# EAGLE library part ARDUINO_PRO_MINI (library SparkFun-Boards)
SparkFun Pro Mini Pro Mini compatible footprint. Dimensions: 0.7 x 1.3" PCB Thickness: 0.8mm SparkFun Products: 3.3V/8MHz 5V/16MHz
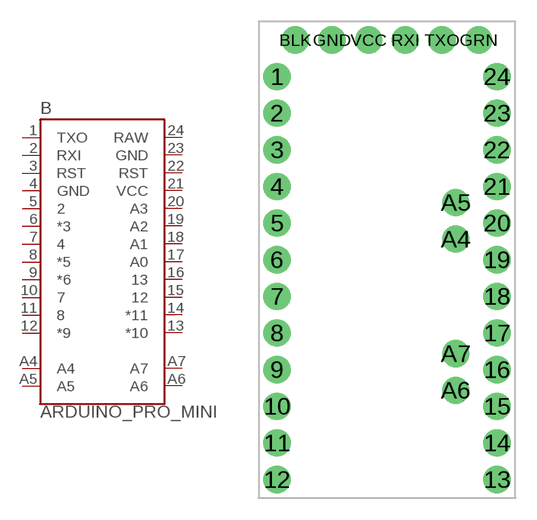
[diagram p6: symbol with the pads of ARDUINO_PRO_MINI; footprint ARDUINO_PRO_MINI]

Designator prefix B

## ARDUINO_PRO_MINI  [ARDUINO_PRO_MINI]
1  TXO
2  RXI
3  RST
4  GND  pwr
5  2
6  *3
7  4
8  *5
9  *6
10  7
11  8
12  *9
13  *10
14  *11
15  12
16  13
17  A0
18  A1
19  A2
20  A3
21  VCC  pwr
22  RST
23  GND  pwr
24  RAW  pwr
A4  A4
A5  A5
A6  A6
A7  A7

## Footprint ARDUINO_PRO_MINI (pad centres in mm)
Arduino Pro Mini Footprint Specifications: Pin count: 34 Area: 1.7 x 0.3 in Example device(s): Arduino Pro Mini
drill 1.016 pad 1.88: 1 -7.62,12.7; 2 -7.62,10.16; 3 -7.62,7.62; 4 -7.62,5.08; 5 -7.62,2.54; 6 -7.62,0; 7 -7.62,-2.54; 8 -7.62,-5.08; 9 -7.62,-7.62; 10 -7.62,-10.16; 11 -7.62,-12.7; 12 -7.62,-15.24; 13 7.62,-15.24; 14 7.62,-12.7; 15 7.62,-10.16; 16 7.62,-7.62; 17 7.62,-5.08; 18 7.62,-2.54; 19 7.62,0; 20 7.62,2.54; 21 7.62,5.08; 22 7.62,7.62; 23 7.62,10.16; 24 7.62,12.7; A4 4.763,1.429; A5 4.763,3.969; A6 4.763,-9.049; A7 4.763,-6.509; BLK -6.35,15.24; GND -3.81,15.24; GRN 6.35,15.24; RXI 1.27,15.24; TXO 3.81,15.24; VCC -1.27,15.24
